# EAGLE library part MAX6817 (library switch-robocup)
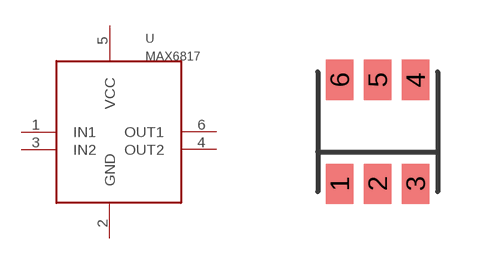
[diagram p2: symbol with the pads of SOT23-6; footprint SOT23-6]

Designator prefix U

## MAX6817  [SOT23-6]
1  IN1
2  GND
3  IN2
4  OUT2
5  VCC
6  OUT1

## Footprint SOT23-6 (pad centres in mm)
smd 0.69 x 1: 1 -0.95,-1.3; 2 0,-1.3; 3 0.95,-1.3; 4 0.95,1.3; 5 0,1.3; 6 -0.95,1.3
